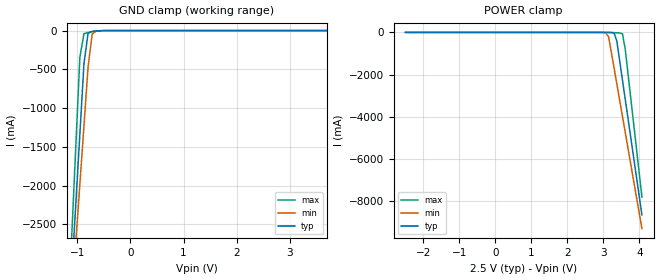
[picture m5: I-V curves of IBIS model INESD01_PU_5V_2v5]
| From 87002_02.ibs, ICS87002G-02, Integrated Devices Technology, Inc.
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[Model] INESD01_PU_5V_2v5
Model_type   Input
Polarity   Non-Inverting
Vinl = .87V
Vinh = 1.62V
|   typ   min   max
C_comp   2pF   1.5pF   2.5pF
|   typ   min   max
[Voltage range]  2.5V   2.375V   2.625V
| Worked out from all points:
|   GND clamp passes 1 mA (typ) near -0.54 V on its own axis
[GND_clamp]
|Voltage   I(typ)   I(min)   I(max)
-1.572V   -8.64A     -8.058A    -9.677A
-1.108V   -3.163A    -3.501A    -2.677A
-1.031V   -2.251A    -2.743A    -1.511A
-953.6mV  -1.339A    -1.985A    -344.3mA
-876.3mV  -427.8mA   -1.227A    -39.97mA
-799mV    -34.67mA   -470.6mA   -24.26mA
-721.6mV  -8.956mA   -46.07mA   -15.49mA
-644.3mV  -3.769mA   -5.089mA   -8.163mA
5V        48.71uA    63.95uA    35.85uA
[POWER_clamp]
|Voltage   I(typ)   I(min)   I(max)
-2.5V     48.71uA    60.9uA     37.74uA
3.067V    -1.276mA   -19.03mA   -266.4uA
3.144V    -3.769mA   -203.7mA   -1.321mA
3.299V    -34.67mA   -1.694A    -10.77mA
3.376V    -427.8mA   -2.452A    -18.7mA
3.531V    -2.251A    -3.969A    -65.35mA
3.608V    -3.163A    -4.728A    -791.3mA
4.072V    -8.64A     -9.287A    -7.79A
